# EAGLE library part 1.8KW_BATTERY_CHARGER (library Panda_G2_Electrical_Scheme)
1.8 kW battery charger
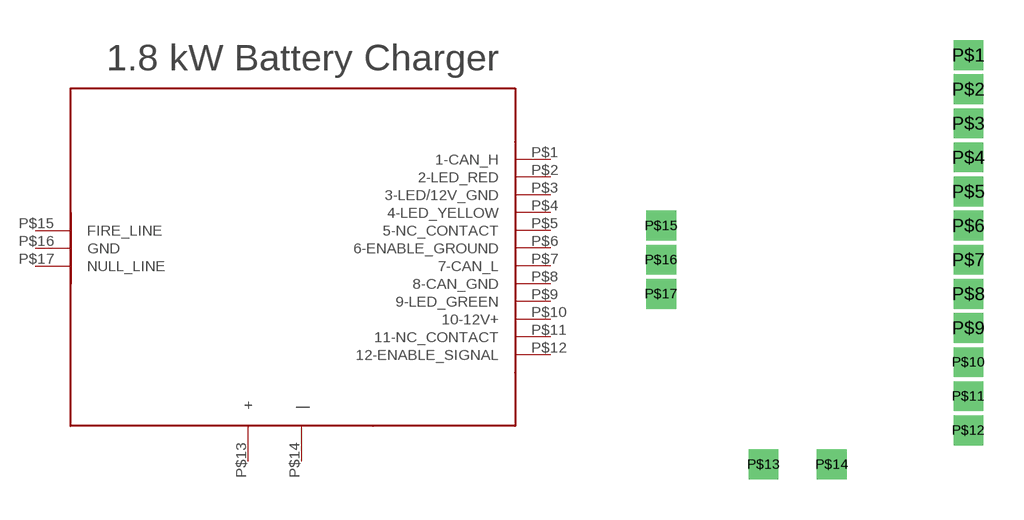
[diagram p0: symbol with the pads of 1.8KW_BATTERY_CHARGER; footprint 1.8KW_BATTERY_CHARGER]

Designator prefix -

## 1.8KW_BATTERY_CHARGER  [1.8KW_BATTERY_CHARGER]
P$1  1-CAN_H
P$2  2-LED_RED
P$3  3-LED/12V_GND
P$4  4-LED_YELLOW
P$5  5-NC_CONTACT
P$6  6-ENABLE_GROUND
P$7  7-CAN_L
P$8  8-CAN_GND
P$9  9-LED_GREEN
P$10  10-12V+
P$11  11-NC_CONTACT
P$12  12-ENABLE_SIGNAL
P$13  +  pwr
P$14  |  pwr
P$15  FIRE_LINE
P$16  GND
P$17  NULL_LINE

## Footprint 1.8KW_BATTERY_CHARGER (pad centres in mm)
drill 0.6 square: P$1 6.35,15.24; P$2 6.35,13.97; P$3 6.35,12.7; P$4 6.35,11.43; P$5 6.35,10.16; P$6 6.35,8.89; P$7 6.35,7.62; P$8 6.35,6.35; P$9 6.35,5.08; P$10 6.35,3.81; P$11 6.35,2.54; P$12 6.35,1.27; P$13 -1.27,0; P$14 1.27,0; P$15 -5.08,8.89; P$16 -5.08,7.62; P$17 -5.08,6.35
